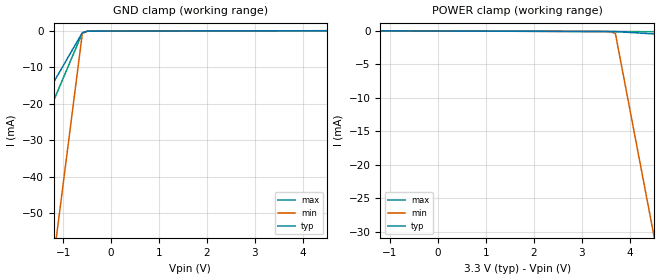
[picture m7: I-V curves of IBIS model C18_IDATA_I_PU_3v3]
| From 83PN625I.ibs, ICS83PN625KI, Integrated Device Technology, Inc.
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[Model] C18_IDATA_I_PU_3v3
Model_type   Input
Polarity   Non-Inverting
Vinl = 0.8V
Vinh = 2.0V
|   typ   min   max
C_comp   2pF   1.5pF   2.5pF
|   typ   min   max
[Voltage range]   3.3V   3.135V   3.465V
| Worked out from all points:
|   GND clamp passes 1 mA (typ) near -0.62 V on its own axis
[GND_clamp]
|Voltage   I (typ)   I (min)   I (max)
-3.3V     -61.84mA   -279.5mA   -84.47mA
-3V       -55.03mA   -248.5mA   -75.15mA
-2.9V     -52.76mA   -238.2mA   -72.04mA
-2.4V     -41.4mA    -186.6mA   -56.51mA
-2.3V     -39.13mA   -176.3mA   -53.41mA
-1.2V     -14.15mA   -62.72mA   -19.24mA
-1.1V     -11.88mA   -52.4mA    -16.13mA
-600mV    -519.6uA   -788.3uA   -601.3uA
-500mV    -121.7uA   -130.5uA   -121.2uA
-400mV    -77.06uA   -71.68uA   -83.32uA
6.6V      65.96uA    64.8uA     66.56uA
[Power_clamp]
|Voltage   I (typ)   I (min)   I (max)
-3.3V     65.96uA    61.71uA    70.06uA
3.5V      -69.96uA   -67.76uA   -74.31uA
3.6V      -72.1uA    -94.44uA   -76.43uA
3.7V      -77.06uA   -368.3uA   -78.55uA
4.4V      -389.3uA   -26.72mA   -94.12uA
4.5V      -433.9uA   -30.49mA   -96.35uA
6.6V      -1.371mA   -109.6mA   -143uA
